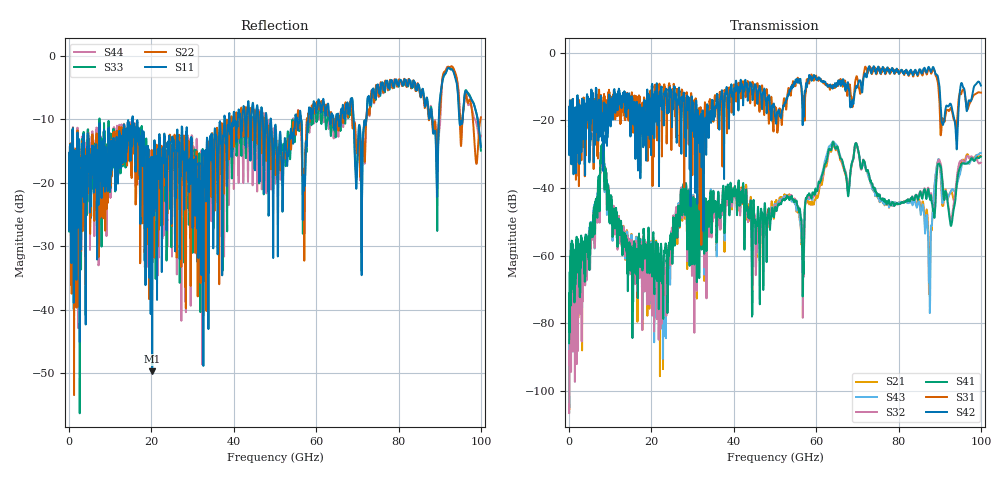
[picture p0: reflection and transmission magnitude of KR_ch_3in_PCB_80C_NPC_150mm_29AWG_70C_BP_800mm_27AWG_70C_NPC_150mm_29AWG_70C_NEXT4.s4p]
# GHz S RI R 45
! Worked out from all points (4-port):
!   4000 points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, 25 MHz to 100 GHz, reference 45 ohm
!   strongest paths, dB at 25 MHz, 25.02 GHz, 50.02 GHz, 75.03 GHz, 100 GHz:
!     S42: -21.8, -20.6, -18.8, -4.2, -9.7
!     S31: -21.7, -12.4, -16.0, -5.0, -11.8
!     S41: -85.8, -60.1, -45.6, -41.8, -30.7
!     S32: -104.0, -53.4, -45.1, -41.8, -32.5
!     S43: -100.6, -56.0, -44.7, -42.8, -29.6
!     S21: -101.5, -55.9, -44.3, -42.9, -30.6
!   lowest |S11| = -49.7 dB at 20.2 GHz (marker M1), VSWR 1.01, Z = 45 - j0.292 ohm
!   |S11| at or under -10 dB: start of sweep to 15.35 GHz; 15.48 GHz to 37.7 GHz (22.22 GHz wide, 83.6 % of centre); 49.02 GHz to 54.9 GHz (5.882 GHz wide, 11.3 % of centre)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
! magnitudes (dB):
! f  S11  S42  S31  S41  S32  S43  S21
! 25 MHz  -17.2  -21.8  -21.7  -85.8  -104.0  -100.6  -101.5
! 8.1 GHz  -13.5  -18.8  -19.0  -29.2  -29.9  -30.0  -29.5
! 20.2 GHz  -49.7  -9.2  -14.2  -66.1  -77.7  -68.0  -70.2
! 56.62 GHz  -15.2  -15.8  -14.0  -59.3  -56.6  -59.1  -57.9
! 64.25 GHz  -10.4  -9.5  -10.1  -26.8  -27.6  -26.3  -27.6
! 87.58 GHz  -9.6  -4.8  -5.0  -42.8  -42.4  -74.7  -63.1
! 100 GHz  -14.3  -9.7  -11.8  -30.7  -32.5  -29.6  -30.6
